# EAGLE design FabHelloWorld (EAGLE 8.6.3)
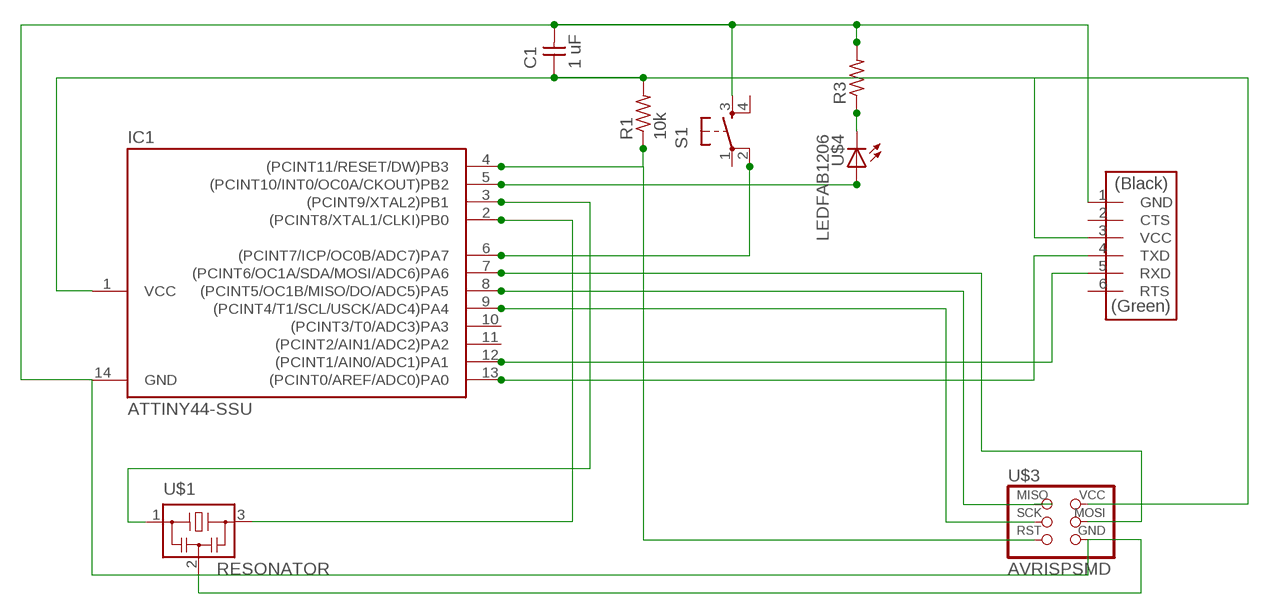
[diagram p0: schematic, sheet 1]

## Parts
C1  1 uF  CAP-UNPOLARIZEDFAB  [C1206FAB]
IC1  ATTINY44-SSU  [SOIC14]
R1  10k  RES-US1206FAB  [R1206FAB]
R3  RES-US1206FAB  [R1206FAB]
S1  6MM_SWITCH6MM_SWITCH  [6MM_SWITCH]
U$1  RESONATOR  [EFOBM]
U$2  FTDI-SMD-HEADER  [1X06SMD]
U$3  AVRISPSMD  [2X03SMD]
U$4  LEDFAB1206  [LED1206FAB]

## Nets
N$1: IC1.6((PCINT7/ICP/OC0B/ADC7)PA7) S1.2(P1)
N$2: IC1.3((PCINT9/XTAL2)PB1) U$1.1
N$3: IC1.2((PCINT8/XTAL1/CLKI)PB0) U$1.3
N$4: C1.1 IC1.1(VCC) R1.2 U$2.3(VCC) U$3.2(VCC)
N$5: IC1.4((PCINT11/RESET/DW)PB3) R1.1 U$3.5(RST)
N$6: IC1.8((PCINT5/OC1B/MISO/DO/ADC5)PA5) U$3.1(MISO)
N$7: IC1.9((PCINT4/T1/SCL/USCK/ADC4)PA4) U$3.3(SCK)
N$8: IC1.7((PCINT6/OC1A/SDA/MOSI/ADC6)PA6) U$3.4(MOSI)
N$9: IC1.13((PCINT0/AREF/ADC0)PA0) U$2.4(TXD)
N$10: IC1.12((PCINT1/AIN0/ADC1)PA1) U$2.5(RXD)
N$11: C1.2 IC1.14(GND) R3.2 S1.3(S) U$1.2 U$2.1(GND) U$3.6(GND)
N$12: IC1.5((PCINT10/INT0/OC0A/CKOUT)PB2) U$4.1(A)
N$13: R3.1 U$4.2(C)
Unconnected: IC1.10((PCINT3/T0/ADC3)PA3) IC1.11((PCINT2/AIN1/ADC2)PA2) S1.1(P) S1.4(S1) U$2.2(CTS) U$2.6(RTS)

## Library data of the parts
C1 = fab:CAP-UNPOLARIZED
IC1 = fab:ATTINY44
R1 R3 = fab:RES-US: Resistor (US Symbol)
S1 = fab:6MM_SWITCH: OMRON SWITCH
U$1 = fab:RESONATOR
U$2 = fab:FTDI-SMD-HEADER
U$3 = fab:AVRISP
U$4 = fab:LED: LED

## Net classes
0 default: clearance 0.402 mm

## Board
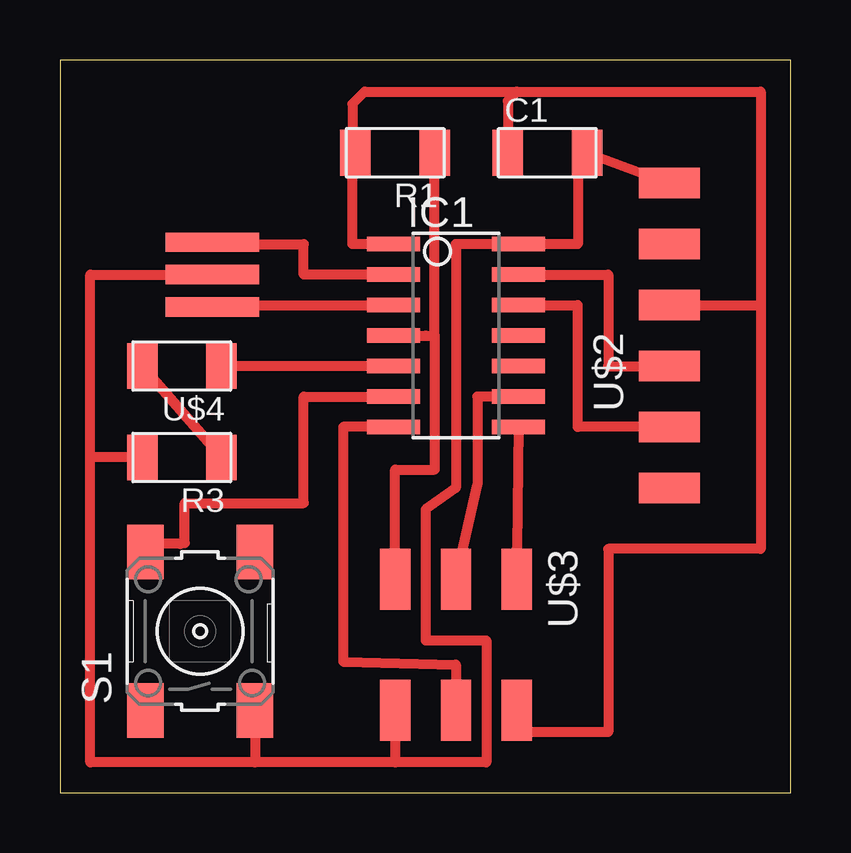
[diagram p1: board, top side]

Size 30.46 x 30.53 mm. Coordinates in mm from the lower left corner, seen from the top.
Outline: 0,0 30.46,0 30.46,30.53 0,30.53 0,0
Copper layers (1*16): Top 0.035mm / dielectric 1.5mm / Bottom 0.035mm
Design rules "FabHelloWorld": minimum track width 6mil, minimum drill 0.35mm, track to track 0.4019mm, track to pad 0.402mm, pad to pad 0.402mm, via to via 0.402mm, smd to smd 6mil, copper to edge 40mil, drill to drill 6mil, minimum pad ring 10mil, minimum via ring 8mil, stop-mask expansion 4mil, vias tented up to drill 0mil, thermal gap 10mil

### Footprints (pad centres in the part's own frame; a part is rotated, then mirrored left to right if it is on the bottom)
C1206FAB = smd 1.27 x 1.905: 1 -1.651,0; 2 1.651,0
SOIC14 = smd 0.61 x 2.21: 1 -3.81,-2.603; 2 -2.54,-2.603; 3 -1.27,-2.603; 4 0,-2.603; 5 1.27,-2.603; 6 2.54,-2.603; 7 3.81,-2.603; 8 3.81,2.603; 9 2.54,2.603; 10 1.27,2.603; 11 0,2.603; 12 -1.27,2.603; 13 -2.54,2.603; 14 -3.81,2.603
R1206FAB = smd 1.27 x 1.905: 1 -1.651,0; 2 1.651,0
6MM_SWITCH = smd 2.286 x 1.524: 1 -3.302,2.286; 2 3.302,2.286; 3 -3.302,-2.286; 4 3.302,-2.286
EFOBM = smd 0.8 x 3.9: 1 -1.35,0; 2 0,0; 3 1.35,0
1X06SMD = smd 2.54 x 1.27: 1 0,6.35; 2 0,3.81; 3 0,1.27; 4 0,-1.27; 5 0,-3.81; 6 0,-6.35
2X03SMD = smd 2.54 x 1.27: 1 -2.54,2.54; 2 2.92,2.54; 3 -2.54,0; 4 2.92,0; 5 -2.54,-2.54; 6 2.92,-2.54
LED1206FAB = smd 1.27 x 1.905: 1 -1.651,0; 2 1.651,0

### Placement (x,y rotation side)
C1  20.32,26.67 0 top
IC1  16.51,19.05 270 top
R1  13.97,26.67 180 top
R3  5.08,13.97 180 top
S1  5.84,6.73 90 top
U$1  6.35,21.59 90 top
U$2  25.4,19.05 0 top
U$3  16.51,6.35 270 top
U$4  5.08,17.78 180 top

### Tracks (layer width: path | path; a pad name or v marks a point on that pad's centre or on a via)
N$1
  Top 0.406: IC1.6 10.16,16.51 10.16,12.06 5.21,12.06 5.21,10.41 5.03,10.37 3.9,10.37 S1.2
N$2
  Top 0.406: IC1.3 6.35,20.32 U$1.1
N$3
  Top 0.406: IC1.2 10.16,21.59 10.16,22.86 6.35,22.86 U$1.3
N$4
  Top 0.406: U$2.3 29.21,20.32 | 29.21,20.32 29.21,10.16 22.86,10.16 22.86,2.54 19.05,2.54 U$3.2 | 29.21,20.32 29.21,29.21 19.05,29.21 | 19.05,29.21 12.7,29.21 12.19,28.7 12.19,26.54 | 19.05,29.21 18.67,28.83 C1.1 | IC1.1 12.19,22.86 12.19,26.54 | 12.19,26.54 R1.2
N$5
  Top 0.406: 15.62,19.05 R1.1 | 15.62,19.05 15.62,13.46 13.97,13.46 U$3.5 | IC1.4 15.24,19.05 15.62,19.05
N$6
  Top 0.406: IC1.8 19.05,10.16 | 19.05,10.16 19.05,9.78 | U$3.1 19.05,10.16
N$7
  Top 0.406: U$3.3 17.4,12.83 17.4,16.51 IC1.9
N$8
  Top 0.406: U$3.4 16.51,5.33 11.81,5.46 11.81,15.24 IC1.7
N$9
  Top 0.406: IC1.13 22.86,21.59 22.86,17.78 U$2.4
N$10
  Top 0.406: IC1.12 21.59,20.32 21.59,15.24 U$2.5
N$11
  Top 0.152: C1.2 21.59,26.29
  Top 0.406: C1.2 U$2.1 | 21.59,26.29 21.59,22.86 IC1.14 16.51,22.86 16.51,12.7 15.24,11.81 15.24,6.35 17.78,6.35 17.78,1.27 13.97,1.27 | 13.97,1.27 8.13,1.27 | 8.13,1.27 1.27,1.27 1.27,13.97 | 1.27,13.97 1.27,21.59 U$1.2 | S1.3 8.13,1.27 | R3.2 1.27,13.97 | U$3.6 13.97,1.27
N$12
  Top 0.406: U$4.1 IC1.5 13.97,17.78
N$13
  Top 0.406: U$4.2 R3.1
